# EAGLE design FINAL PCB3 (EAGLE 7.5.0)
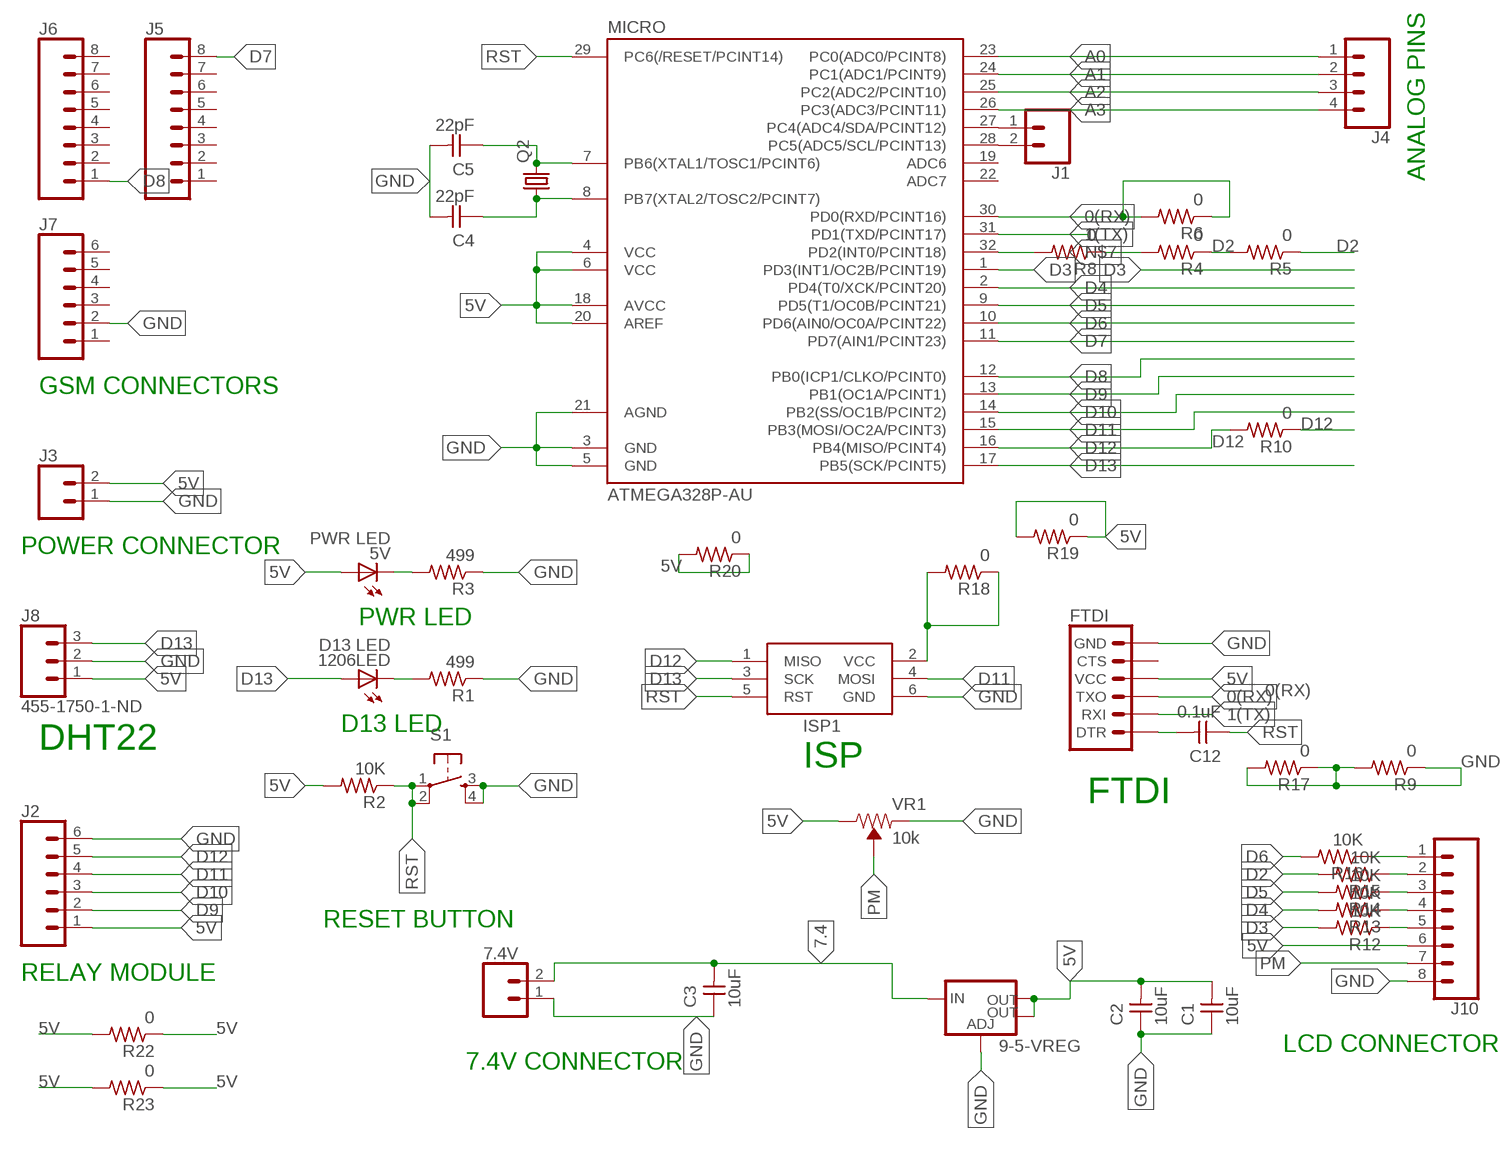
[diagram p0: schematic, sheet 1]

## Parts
5V  PWR LED  LEDFAB1206  [LED1206FAB]
7.4V  CONN_02LOCK  [1X02_LOCK]
9-5-VREG  V_REG_LM1117SOT223  [SOT223]
1206LED  D13 LED  LEDFAB1206  [LED1206FAB]
C1  10uF  CAP-UNPOLARIZEDFAB  [C1206FAB]
C2  10uF  CAP-UNPOLARIZEDFAB  [C1206FAB]
C3  10uF  CAP-UNPOLARIZEDFAB  [C1206FAB]
C4  22pF  CAP-UNPOLARIZEDFAB  [C1206FAB]
C5  22pF  CAP-UNPOLARIZEDFAB  [C1206FAB]
C12  0.1uF  CAP-UNPOLARIZEDFAB  [C1206FAB]
FTDI  6_PIN_SERIAL_TARGET_SILK  [1X06]
ISP1  AVRISP-6  [AVRISP]
J1  CONN_02  [1X02]
J2  CONN_06SILK_FEMALE_PTH  [1X06]
J3  CONN_02  [1X02]
J4  CONN_04  [1X04]
J5  CONN_08"  [1X08]
J6  CONN_08"  [1X08]
J7  CONN_06SILK_FEMALE_PTH  [1X06]
J8  455-1750-1-ND  CONN_03  [1X03]
J10  CONN_08"  [1X08]
MICRO  ATMEGA328P-AU  ATMEGA48/88/168-AU  [TQFP32-08]
Q2  CRYSTALHC49U70  [HC49U70]
R1  499  RES-US1206FAB  [R1206FAB]
R2  10K  RES-US1206FAB  [R1206FAB]
R3  499  RES-US1206FAB  [R1206FAB]
R4  0  RES-US1206FAB  [R1206FAB]
R5  0  RES-US1206FAB  [R1206FAB]
R6  0  RES-US1206FAB  [R1206FAB]
R8  0  RES-US1206FAB  [R1206FAB]
R9  0  RES-US1206FAB  [R1206FAB]
R10  0  RES-US1206FAB  [R1206FAB]
R12  10K  RES-US1206FAB  [R1206FAB]
R13  10K  RES-US1206FAB  [R1206FAB]
R14  10K  RES-US1206FAB  [R1206FAB]
R15  10K  RES-US1206FAB  [R1206FAB]
R16  10K  RES-US1206FAB  [R1206FAB]
R17  0  RES-US1206FAB  [R1206FAB]
R18  0  RES-US1206FAB  [R1206FAB]
R19  0  RES-US1206FAB  [R1206FAB]
R20  0  RES-US1206FAB  [R1206FAB]
R22  0  RES-US1206FAB  [R1206FAB]
R23  0  RES-US1206FAB  [R1206FAB]
S1  6MM_SWITCH6MM_SWITCH  [6MM_SWITCH]
VR1  10k  TRIMPOT-PTH-10MM-KNOB-1/2W-10%  [TRIMPOT-PTH-3386U]

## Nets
0(RX): FTDI.3(TXO) MICRO.30(PD0(RXD/PCINT16)) R6.1 R6.2
1(TX): FTDI.2(RXI) MICRO.31(PD1(TXD/PCINT17))
5V: 5V.1(A) 9-5-VREG.2(OUT) 9-5-VREG.4(OUT) C1.2 C2.2 FTDI.4(VCC) ISP1.2(VCC) J2.1 J3.2 J8.1 J10.6 MICRO.4(VCC) MICRO.6(VCC) MICRO.18(AVCC) MICRO.20(AREF) R2.2 R18.1 R18.2 R19.1 R19.2 R20.1 R20.2 R22.1 R22.2 R23.1 R23.2 VR1.3(CW)
7.4: 7.4V.2 9-5-VREG.3(IN) C3.2
A0: J4.1 MICRO.23(PC0(ADC0/PCINT8))
A1: J4.2 MICRO.24(PC1(ADC1/PCINT9))
A2: J4.3 MICRO.25(PC2(ADC2/PCINT10))
A3: J4.4 MICRO.26(PC3(ADC3/PCINT11))
D2: R4.1 R4.2 R5.1 R5.2 R8.1 R15.2
D3: MICRO.1(PD3(INT1/OC2B/PCINT19)) R12.2
D4: MICRO.2(PD4(T0/XCK/PCINT20)) R13.2
D5: MICRO.9(PD5(T1/OC0B/PCINT21)) R14.2
D6: MICRO.10(PD6(AIN0/OC0A/PCINT22)) R16.2
D7: J5.8 MICRO.11(PD7(AIN1/PCINT23))
D8: J6.1 MICRO.12(PB0(ICP1/CLKO/PCINT0))
D9: J2.2 MICRO.13(PB1(OC1A/PCINT1))
D10: J2.3 MICRO.14(PB2(SS/OC1B/PCINT2))
D11: ISP1.4(MOSI) J2.4 MICRO.15(PB3(MOSI/OC2A/PCINT3))
D12: ISP1.1(MISO) J2.5 MICRO.16(PB4(MISO/PCINT4)) R10.1 R10.2
D13: 1206LED.1(A) ISP1.3(SCK) J8.3 MICRO.17(PB5(SCK/PCINT5))
GND: 7.4V.1 9-5-VREG.1(ADJ) C1.1 C2.1 C3.1 C4.2 C5.2 FTDI.6(GND) ISP1.6(GND) J2.6 J3.1 J7.2 J8.2 J10.8 MICRO.3(GND) MICRO.5(GND) MICRO.21(AGND) R1.1 R3.1 R9.1 R9.2 R17.1 R17.2 S1.3(S) S1.4(S1) VR1.1(CCW)
N$1: 1206LED.2(C) R1.2
N$2: 5V.2(C) R3.2
N$3: C5.1 MICRO.7(PB6(XTAL1/TOSC1/PCINT6)) Q2.2
N$4: C4.1 MICRO.8(PB7(XTAL2/TOSC2/PCINT7)) Q2.1
N$7: MICRO.32(PD2(INT0/PCINT18)) R8.2
N$8: J1.1 MICRO.27(PC4(ADC4/SDA/PCINT12))
N$9: J1.2 MICRO.28(PC5(ADC5/SCL/PCINT13))
N$13: J10.5 R12.1
N$14: J10.4 R13.1
N$15: J10.3 R14.1
N$16: C12.2 FTDI.1(DTR)
N$17: J10.2 R15.1
N$18: J10.1 R16.1
PM: J10.7 VR1.2(WIPER)
RST: C12.1 ISP1.5(RST) MICRO.29(PC6(/RESET/PCINT14)) R2.1 S1.1(P) S1.2(P1)
Unconnected: FTDI.5(CTS) J5.1 J5.2 J5.3 J5.4 J5.5 J5.6 J5.7 J6.2 J6.3 J6.4 J6.5 J6.6 J6.7 J6.8 J7.1 J7.3 J7.4 J7.5 J7.6 MICRO.19(ADC6) MICRO.22(ADC7)

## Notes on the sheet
- ANALOG PINS
- GSM CONNECTORS
- POWER CONNECTOR
- PWR LED
- D13 LED
- DHT22
- ISP
- FTDI
- RESET BUTTON
- RELAY MODULE
- LCD CONNECTOR
- 7.4V CONNECTOR

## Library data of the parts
5V 1206LED = fab:LED: LED
7.4V J1 J3 = SparkFun-Connectors:CONN_02: Multi connection point. Often used as Generic Header-pin footprint for 0.1 inch spaced/style header connections
9-5-VREG = fab:V_REG_LM1117: Voltage Regulator LM1117 Standard adjustable voltage regulator but in SMD form. Spark Fun Electronics SKU : COM-00595; PROD_ID: VREG-08170
C1-C5 C12 = fab:CAP-UNPOLARIZED
FTDI = SparkFun-Connectors:6_PIN_SERIAL_TARGET: 6-pin header connection for use with the "FTDI BASIC" pinout - TARGET SIDE. Also known as "Arduino Serial Program Header". It is used to mate with our FTDI Basic serial programmers using the Arduino IDE. Note, this device has "TARGET" in the name. It is intended to be used on a design that contains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
ISP1 = adafruit:AVRISP: AVR ISP HEADER Standard 6 pin header for AVR programming
J2 J7 = SparkFun-Connectors:CONN_06: Multi connection point. Often used as Generic Header-pin footprint for 0.1 inch spaced/style header connections On any of the 0.1 inch spaced packages, you can populate with these: Break Away Headers - Straight (PRT-00116) Break Away Male Headers - Right Angle (PRT-00553) Female Headers (PRT-00115)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; PROD_ID: CONN-08437
J4 = SparkFun-Connectors:CONN_04: Multi connection point. Often used as Generic Header-pin footprint for 0.1 inch spaced/style header connections On any of the 0.1 inch spaced packages, you can populate with these: Break Away Headers - Straight (PRT-00116) Break Away Male Headers - Right Angle (PRT-00553) Female Headers (PRT-00115)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; PROD_ID: CONN-09696
J5 J6 J10 = SparkFun-Connectors:CONN_08: Multi connection point. Often used as Generic Header-pin footprint for 0.1 inch spaced/style header connections On any of the 0.1 inch spaced packages, you can populate with these: Break Away Headers - Straight (PRT-00116) Break Away Male Headers - Right Angle (PRT-00553) Female Headers (PRT-00115)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; PROD_ID: CONN-08438
J8 = SparkFun-Connectors:CONN_03: Multi connection point. Often used as Generic Header-pin footprint for 0.1 inch spaced/style header connections On any of the 0.1 inch spaced packages, you can populate with these: Break Away Headers - Straight (PRT-00116) Break Away Male Headers - Right Angle (PRT-00553) Female Headers (PRT-00115)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; PROD_ID: XXX-00000
MICRO = atmega8:ATMEGA48/88/168
Q2 = crystal:CRYSTAL: CRYSTAL; OC_FARNELL: unknown; OC_NEWARK: unknown
R1-R6 R8-R10 R12-R20 R22 R23 = fab:RES-US: Resistor (US Symbol)
S1 = fab:6MM_SWITCH: OMRON SWITCH
VR1 = SparkFun-Resistors:TRIMPOT: Trimming Potentiometer (Trimpot) Three-terminal potentiometers, with an adjustable wiper and two adjustable resistors. A pot can be used to create a configurable voltage divider, or as a variable resistor. "Trimpots" are a subset of potentiometers, usually intended for "set-and-forget"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; PROD_ID: RES-09730; SF_SKU: COM-09806

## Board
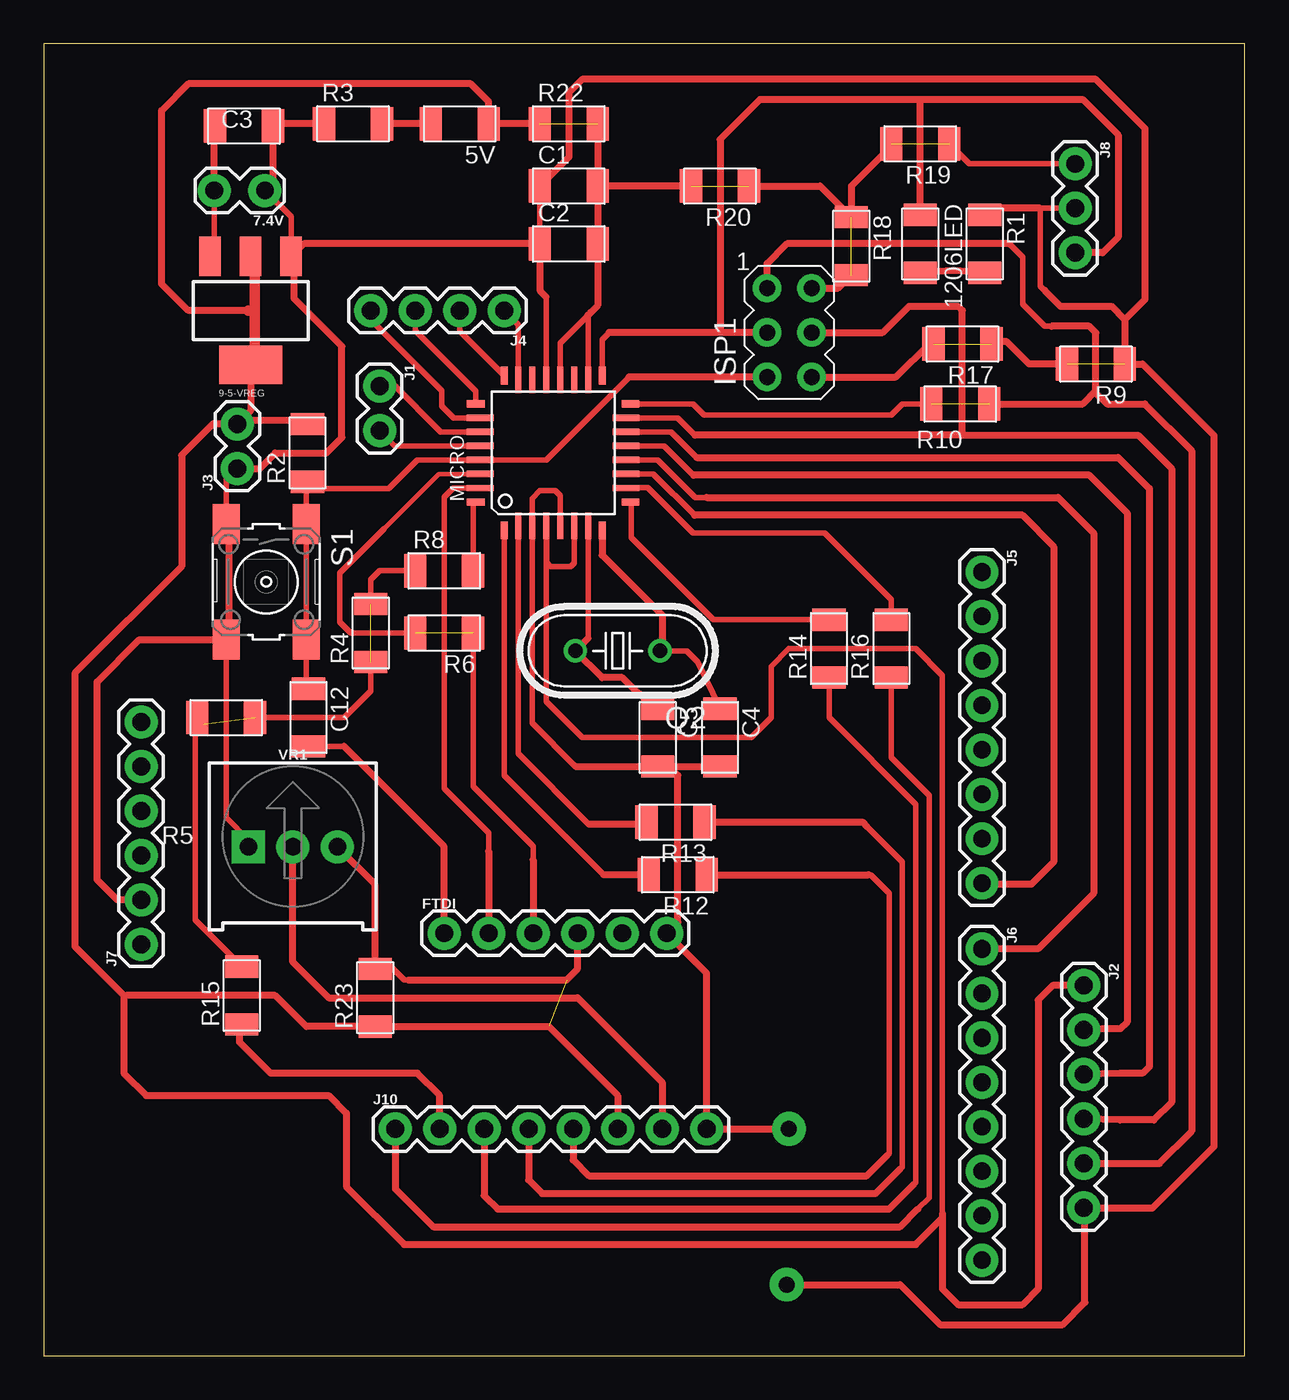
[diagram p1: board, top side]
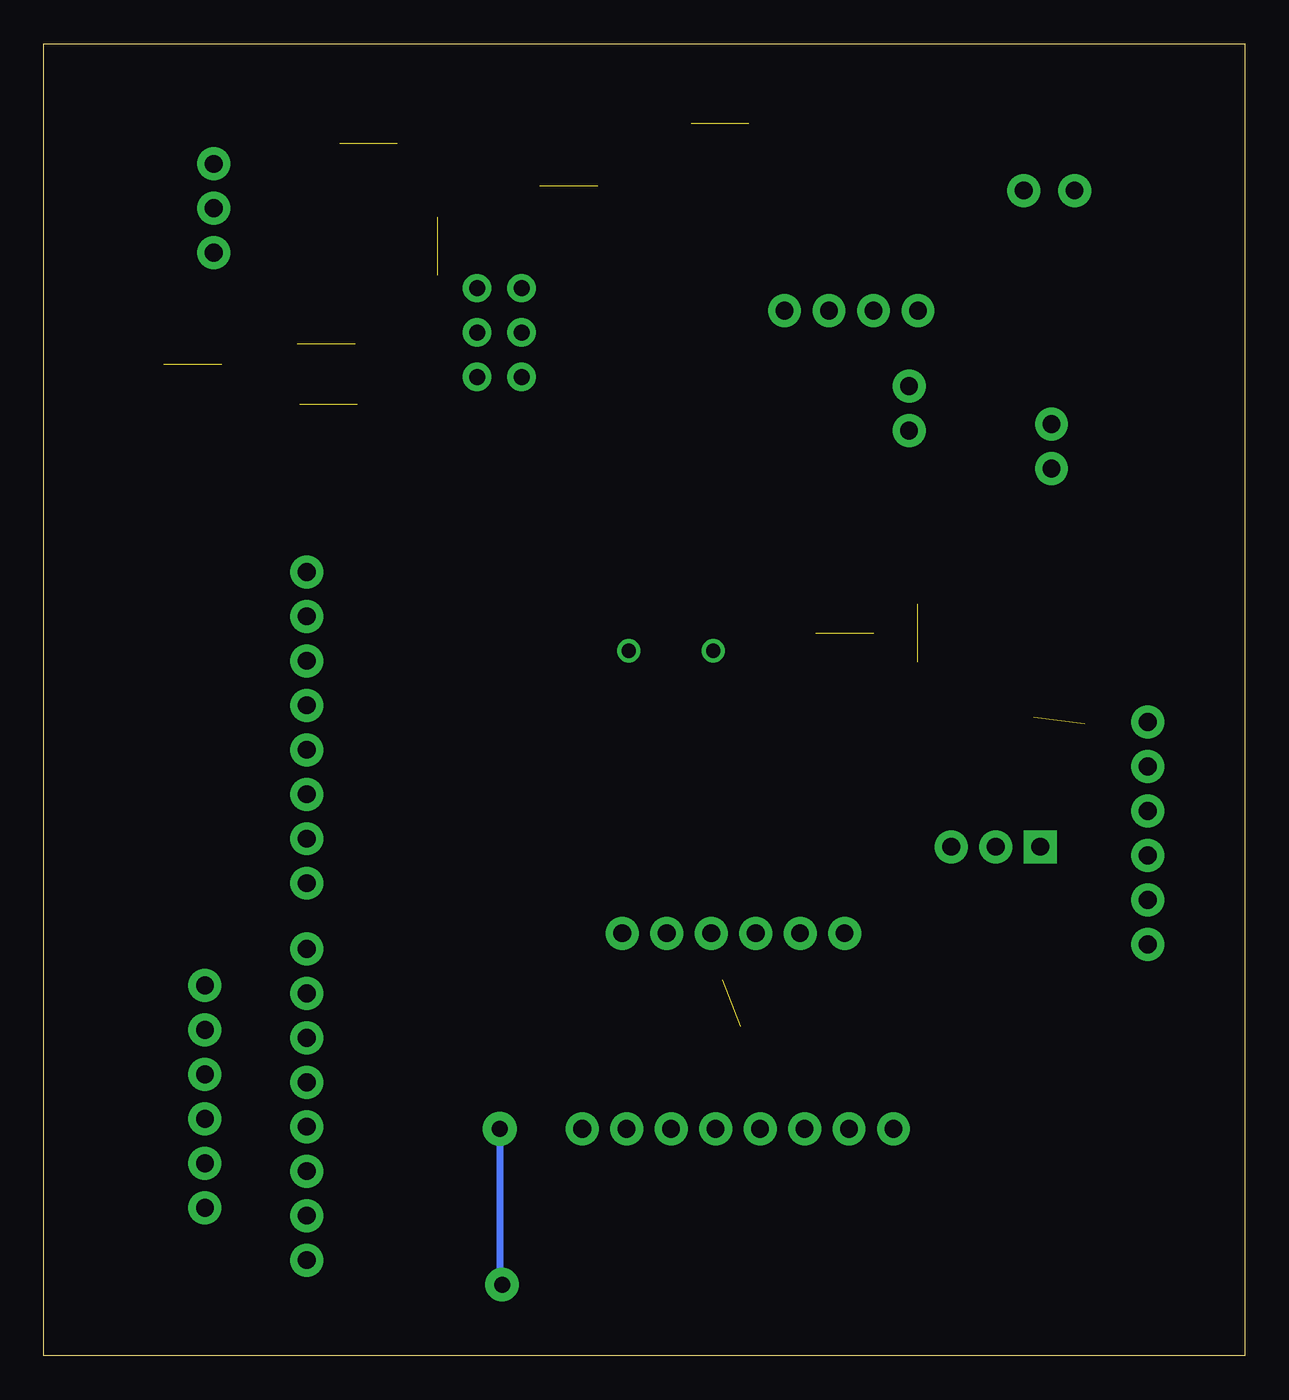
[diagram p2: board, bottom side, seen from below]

Size 68.58 x 74.93 mm. Coordinates in mm from the lower left corner, seen from the top.
Outline: 0,0 68.58,0 68.58,74.93 0,74.93 0,0
Copper layers (1*16): Top 0.035mm / dielectric 1.5mm / Bottom 0.035mm
Design rules "default *": minimum track width 10mil, minimum drill 24mil, track to track 12mil, track to pad 12mil, pad to pad 12mil, via to via 12mil, smd to smd 8mil, copper to edge 40mil, drill to drill 8mil, minimum pad ring 10mil, minimum via ring 8mil, stop-mask expansion 4mil, vias tented up to drill 0mil, thermal gap 10mil

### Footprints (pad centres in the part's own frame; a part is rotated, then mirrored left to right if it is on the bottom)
LED1206FAB = smd 1.27 x 1.905: 1 -1.651,0; 2 1.651,0
1X02_LOCK = drill 1.016 pad 1.88: 1 -0.178,0; 2 2.718,0
SOT223 = smd 1.219 x 2.235: 1 -2.311,-3.099; 2 0,-3.099; 3 2.311,-3.099 | smd 3.6 x 2.2: 4 0,3.099
C1206FAB = smd 1.27 x 1.905: 1 -1.651,0; 2 1.651,0
1X06 = drill 1.016 pad 1.88: 1 0,0; 2 2.54,0; 3 5.08,0; 4 7.62,0; 5 10.16,0; 6 12.7,0
AVRISP = drill 0.9 pad 1.626: 1 -1.27,2.54; 2 1.27,2.54; 3 -1.27,0; 4 1.27,0; 5 -1.27,-2.54; 6 1.27,-2.54
1X02 = drill 1.016 pad 1.88: 1 0,0; 2 2.54,0
1X04 = drill 1.016 pad 1.88: 1 0,0; 2 2.54,0; 3 5.08,0; 4 7.62,0
1X08 = drill 1.016 pad 1.88: 1 0,0; 2 2.54,0; 3 5.08,0; 4 7.62,0; 5 10.16,0; 6 12.7,0; 7 15.24,0; 8 17.78,0
1X03 = drill 1.016 pad 1.88: 1 0,0; 2 2.54,0; 3 5.08,0
TQFP32-08 = smd 1.016 x 0.406: 1 -4.42,2.8; 8 -4.42,-2.8; 17 4.42,-2.8; 24 4.42,2.8 | smd 1.524 x 0.356: 2 -4.166,2; 3 -4.166,1.2; 4 -4.166,0.4; 5 -4.166,-0.4; 6 -4.166,-1.2; 7 -4.166,-2; 18 4.166,-2; 19 4.166,-1.2; 20 4.166,-0.4; 21 4.166,0.4; 22 4.166,1.2; 23 4.166,2 | smd 0.406 x 1.016: 9 -2.8,-4.42; 16 2.8,-4.42; 25 2.8,4.42; 32 -2.8,4.42 | smd 0.356 x 1.524: 10 -2,-4.166; 11 -1.2,-4.166; 12 -0.4,-4.166; 13 0.4,-4.166; 14 1.2,-4.166; 15 2,-4.166; 26 2,4.166; 27 1.2,4.166; 28 0.4,4.166; 29 -0.4,4.166; 30 -1.2,4.166; 31 -2,4.166
HC49U70 = drill 0.813: 1 -2.413,0; 2 2.413,0
R1206FAB = smd 1.27 x 1.905: 1 -1.651,0; 2 1.651,0
6MM_SWITCH = smd 2.286 x 1.524: 1 -3.302,2.286; 2 3.302,2.286; 3 -3.302,-2.286; 4 3.302,-2.286
TRIMPOT-PTH-3386U = drill 1.016 pad 1.88 square: 1 -2.54,-0.015 | drill 1.016 pad 1.88: 2 0,-0.015; 3 2.54,-0.015

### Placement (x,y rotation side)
5V  23.75,70.36 180 top
7.4V  12.45,66.55 180 top
9-5-VREG  11.81,59.69 180 top
1206LED  50.04,63.5 270 top
C1  29.97,66.8 0 top
C2  29.97,63.5 0 top
C3  11.43,70.23 180 top
C4  38.61,35.31 270 top
C5  35.05,35.31 270 top
C12  15.11,36.45 270 top
FTDI  22.86,24.13 0 top
ISP1  42.57,58.43 0 top
J1  19.18,55.37 270 top
J2  59.38,21.15 270 top
J3  11.05,50.67 90 top
J4  26.29,59.69 180 top
J5  53.56,44.77 270 top
J6  53.56,23.24 270 top
J7  5.56,23.5 90 top
J8  58.88,68.07 270 top
J10  20.07,12.95 0 top
MICRO  29.08,51.56 90 top
Q2  32.77,40.26 180 top
R1  53.72,63.5 270 top
R2  15.05,51.56 90 top
R3  17.65,70.36 0 top
R4  18.67,41.27 90 top
R5  10.41,36.45 0 top
R6  22.86,41.27 180 top
R8  22.86,44.83 0 top
R9  60.07,56.64 180 top
R10  52.32,54.36 180 top
R12  36.2,27.47 180 top
R13  36.07,30.47 180 top
R14  44.83,40.39 90 top
R15  11.3,20.57 90 top
R16  48.39,40.39 90 top
R17  52.45,57.78 180 top
R18  46.1,63.37 270 top
R19  50.04,69.22 180 top
R20  38.61,66.8 180 top
R22  29.97,70.36 0 top
R23  18.92,20.45 90 top
S1  12.7,44.2 270 top
VR1  14.22,29.08 0 top

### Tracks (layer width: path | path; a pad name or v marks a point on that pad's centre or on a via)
0(RX)  (1 unrouted)
  Top 0.254: 19.43,47.24 22.55,50.36 MICRO.30
  Top 0.305: 27.94,28.32 27.94,29.08 24.51,32.51 R6.1 | R6.2 17.53,41.27 16.89,41.91 16.89,44.7 19.43,47.24
  Top 0.406: 27.94,28.32 FTDI.3
1(TX)
  Top 0.305: MICRO.31 23.37,49.56 22.86,49.05 22.86,32.38 25.4,29.84 25.4,28.83
  Top 0.406: 25.4,28.83 FTDI.2
5V  (5 unrouted)
  Top 0.254: 11.91,62.66 9-5-VREG.2 12.04,62.64 | 11.91,56.79 11.83,56.63 9-5-VREG.4 | 12.04,56.77 9-5-VREG.4 | 14.88,53.42 R2.2 | 11.76,56.49 9-5-VREG.4
  Top 0.305: 11.81,56.63 11.83,56.63 | MICRO.20 29.48,57.84 31.08,59.44 MICRO.18 | 20.83,21.46 20.57,21.46 19.81,22.23 19.05,22.23 R23.2 | MICRO.6 30.28,45.27 30.1,45.09 28.96,45.09 28.7,45.34 28.7,47.38 MICRO.4 28.68,37.36 30.73,35.31 40.39,35.31 41.53,36.45 41.53,39.37 42.55,40.39 49.78,40.39 51.31,38.86 51.31,8.13 51.31,7.87 | J8.1 52.83,68.07 R19.1 | 12.04,56.82 9-5-VREG.4
  Top 0.406: ISP1.2 45.35,60.97 R18.2 | 11.68,59.69 8.26,59.69 6.73,61.21 6.73,71.12 8.26,72.64 24.38,72.64 25.4,71.63 5V.1 R22.1 | 31.08,59.44 31.23,59.58 31.62,59.98 C2.2 C1.2 | R20.1 44.32,66.8 R18.1 46.1,66.8 48.39,69.09 R19.2 | R20.2 C1.2 | R22.2 C1.2 | R23.2 18.92,26.91 VR1.3 | 20.83,21.46 29.84,21.46 30.48,22.1 FTDI.4 | 51.31,8.13 51.31,3.81 52.2,2.92 55.88,2.92 56.77,3.81 56.77,20.32 57.6,21.15 J2.1 | J10.6 32.77,14.86 28.83,18.8 R23.1 14.99,18.8 13.21,20.57 4.7,20.57 4.57,20.45 | 9-5-VREG.4 11.81,53.98 11.25,53.42 | 11.25,53.42 J3.2 9.65,53.21 7.87,51.44 7.87,45.09 1.78,38.99 1.78,23.37 4.57,20.57 4.57,20.45 | 14.88,53.42 11.25,53.42 | 4.57,20.45 4.57,16.13 5.84,14.86 16.26,14.86 17.27,13.84 17.27,9.65 20.57,6.35 49.78,6.35 51.31,7.87
  Top 0.61: 12.04,62.64 12.04,59.69 | 12.04,59.69 12.04,56.82 | 11.68,59.69 12.04,59.69
7.4
  Top 0.254: 9.73,62.98 9-5-VREG.3
  Top 0.305: 9-5-VREG.3 9.73,62.79 7.4V.2
  Top 0.406: 7.4V.2 9.73,70.18 C3.2
A0
  Top 0.305: MICRO.23 27.08,58.9 J4.1
A1
  Top 0.305: J4.2 23.75,58.52 MICRO.24
A2
  Top 0.305: MICRO.25 24.66,55.09 21.21,58.55 J4.3
A3
  Top 0.305: J4.4 18.67,59.18 22.73,55.12 22.73,54.23 23.4,53.56 MICRO.26
D2  (2 unrouted)
  Top 0.305: R5.2 17.14,36.45 18.67,37.97 R4.1 | R8.1 19.18,44.83 18.67,44.32 R4.2 | 8.64,36.32 8.64,24.89 R15.2
  Top 0.406: 9.14,36.07 R5.1 8.64,36.32
D3
  Top 0.305: MICRO.1 26.28,33.15 31.96,27.47
  Top 0.406: R12.2 31.96,27.47
D4
  Top 0.305: MICRO.2 27.08,34.38 31.11,30.35
  Top 0.406: R13.2 34.29,30.35 31.11,30.35
D5
  Top 0.254: 33.5,48.74 MICRO.9
  Top 0.305: R14.2 38.23,42.04 33.53,46.74 33.53,48.74 MICRO.9
D6
  Top 0.254: 33.5,49.58 MICRO.10
  Top 0.305: 33.5,49.58 34.49,49.58 37.08,46.99 44.58,46.99 48.39,43.18 R16.2
D7
  Top 0.305: MICRO.11 34.8,50.36 37.15,48.01
  Top 0.406: 37.15,48.01 55.88,48.01 57.66,46.23 57.66,28.19 56.39,26.92 53.63,26.92 J5.8
D8
  Top 0.305: MICRO.12 35.05,51.16 37.19,49.02 37.85,49.02
  Top 0.406: 37.85,49.02 57.91,49.02 59.94,46.99 59.94,26.42 56.77,23.24 J6.1
D9
  Top 0.305: MICRO.13 33.27,51.94 35.43,51.94 37.08,50.29
  Top 0.406: 37.08,50.29 59.69,50.29 61.85,48.13 61.85,19.05 61.47,18.67 60.44,18.67 J2.2
D10
  Top 0.305: MICRO.14 35.81,52.76 37.27,51.31
  Top 0.406: 37.27,51.31 61.34,51.31 63.12,49.53 63.12,16.51 62.74,16.13 61.44,16.13 J2.3
D11
  Top 0.305: MICRO.15 36.2,53.56 37.18,52.58
  Top 0.406: 52.45,52.58 52.45,59.69 52.2,59.94 49.4,59.94 47.89,58.43 ISP1.4 | 52.45,52.58 37.18,52.58 | 52.45,52.58 62.48,52.58 64.39,50.67 64.39,14.48 63.37,13.46 61.45,13.46 J2.4
D12  (1 unrouted)
  Top 0.305: R10.2 49.02,54.36 48.39,53.72 37.72,53.72 37.08,54.36 MICRO.16 | 57.53,58.8 57.15,58.8 55.88,60.07 55.88,62.74 55.12,63.5
  Top 0.406: 55.12,63.5 42.42,63.5 41.3,62.38 ISP1.1 | R10.1 59.31,54.36 60.07,55.12 | 60.07,55.12 60.07,58.42 59.69,58.8 57.53,58.8 | 60.07,55.12 60.07,54.99 60.71,54.36 62.87,54.36 65.53,51.69 65.53,12.83 63.69,10.99 J2.5
D13
  Top 0.305: MICRO.17 31.88,58.04 32.28,58.43
  Top 0.406: ISP1.3 38.48,58.43 | 38.48,58.43 32.28,58.43 | 38.48,58.43 38.61,58.56 38.61,69.47 40.89,71.75 50.16,71.75 | J8.3 60.45,62.99 61.34,63.88 61.34,69.72 59.31,71.75 50.16,71.75 | 1206LED.1 50.04,71.63 50.16,71.75
GND  (via drill 0.91 pad 1.93)  (2 unrouted)
  Top 0.254: 14.25,62.97 9-5-VREG.1 14.28,62.92 | 28.7,55.78 MICRO.21 | 28.7,55.5 MICRO.21 | 10.57,41 S1.4 | 10.57,47.42 S1.3 | MICRO.21 28.75,55.73
  Top 0.305: J3.1 10.41,50.04 S1.3 | MICRO.3 27.88,48.97 28.32,49.4 29.21,49.4 29.48,49.13 MICRO.5 | MICRO.3 27.91,47.4 27.91,47.35 | 28.68,60.47 MICRO.21 | 7.4V.1 14.12,65.05 9-5-VREG.1 | VR1.1 11.68,29.46 10.41,30.73 S1.4 | C1.1 C2.1 | 57.15,60.83 56.9,61.09 56.9,65.53 J8.2 | MICRO.3 27.88,36.12 30.35,33.66
  Top 0.406: 35.69,33.66 C5.2 30.35,33.66 | 35.69,33.66 C4.2 | ISP1.6 48.66,55.89 50.55,57.78 R17.2 | VR1.1 12.19,28.56 | 9-5-VREG.1 14.83,63.5 C2.1 28.32,60.83 28.68,60.47 | 14.28,62.92 14.28,60.4 17.02,57.66 17.02,52.45 16.13,51.56 13.21,51.56 12.32,50.67 J3.1 | J7.2 4.19,26.04 3.05,27.18 3.05,38.48 5.46,40.89 S1.4 10.57,41.05 10.57,47.42 | 57.15,60.83 58.04,59.94 60.96,59.94 61.72,59.18 | 56.9,65.53 54.1,65.53 R1.1 | R9.2 56.26,56.64 54.99,57.91 54.23,57.91 R17.1 | C1.1 29.97,68.45 29.97,72.14 30.73,72.9 60.07,72.9 62.87,70.1 62.87,60.33 61.72,59.18 | R3.1 13.21,70.36 C3.1 13.08,67 7.4V.1 | 35.69,33.66 36.2,33.15 36.2,24.77 FTDI.6 37.85,21.84 J10.8 v42.55,12.95 | v42.42,4.06 48.9,4.06 51.18,1.78 58.17,1.78 59.44,3.05 59.44,8.39 J2.6 63.31,8.45 66.8,11.94 66.8,52.58 62.74,56.64 R9.1 61.72,59.18
  Bottom 0.406: v42.55,12.95 42.55,4.19 v42.42,4.06
N$1
  Top 0.406: R1.2 51.94,61.98 1206LED.2
N$2
  Top 0.406: 5V.2 R3.2
N$3
  Top 0.305: MICRO.7 31.08,40.99
  Top 0.406: C5.1 33.91,37.85 33.02,38.73 31.88,38.73 Q2.2 30.86,40.77 31.08,40.99
N$4
  Top 0.254: 31.83,47.07 MICRO.8
  Top 0.305: C4.1 37.34,39.62 36.7,40.26 Q2.1 34.8,40.26 | MICRO.8
  Top 0.406: MICRO.8 31.88,45.72 35.31,42.29 35.31,40.39 Q2.1
N$7
  Top 0.254: 24.84,48.74 MICRO.32
  Top 0.305: R8.2 24.51,48.61 MICRO.32
N$8
  Top 0.305: MICRO.27 22.68,52.76 19.94,55.5 19.3,55.5 J1.1
N$9
  Top 0.305: MICRO.28 20.05,51.96 J1.2
N$13
  Top 0.305: 48.13,11.43 48.26,11.56 48.26,26.42 47.2,27.47 47.08,27.47
  Top 0.406: J10.5 30.23,11.18 31.11,10.29 46.99,10.29 48.13,11.43 | R12.1 47.08,27.47
N$14
  Top 0.305: 46.99,30.23 49.02,28.19 49.02,10.79 48.9,10.67
  Top 0.406: J10.4 27.69,10.03 28.45,9.27 47.5,9.27 48.9,10.67 | R13.1 46.74,30.47 46.99,30.23
N$15
  Top 0.305: R14.1 44.83,36.45 49.78,31.5 49.78,9.91 49.66,9.78
  Top 0.406: J10.3 25.15,9.14 25.91,8.38 48.26,8.38 49.66,9.78
N$16
  Top 0.305: 17.14,34.8 C12.2
  Top 0.406: FTDI.1 22.86,29.08 17.14,34.8
N$17
  Top 0.406: J10.2 22.61,14.86 21.34,16.13 12.95,16.13 11.18,17.91 11.18,18.8 R15.1
N$18
  Top 0.305: R16.1 48.39,34.16 50.55,32 50.55,9.02 49.91,8.38
  Top 0.406: J10.1 20.07,9.53 22.23,7.37 48.9,7.37 49.91,8.38
PM
  Top 0.406: VR1.2 14.22,22.48 16.26,20.45 30.48,20.45 35.31,15.62 J10.7
RST
  Top 0.254: 15.09,37.87 C12.1 15.16,38.15 | 15.04,40.72 S1.2 15.04,41 | 15.62,50.06 15.35,50.15 R2.1 15.16,49.78
  Top 0.305: 15.62,49.53 15.62,50.06 | C12.1 14.99,38.23 S1.2 S1.1 14.99,49.53 15.62,49.53 | 15.62,49.53 19.7,49.53 21.34,51.16 MICRO.29 28.68,51.16 33.41,55.89
  Top 0.406: ISP1.5 33.41,55.89

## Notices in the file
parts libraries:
SparkFun-Connectors: Licensing: Creative Commons ShareAlike 4.0 International - https://creativecommons.org/licenses/by-sa/4.0
